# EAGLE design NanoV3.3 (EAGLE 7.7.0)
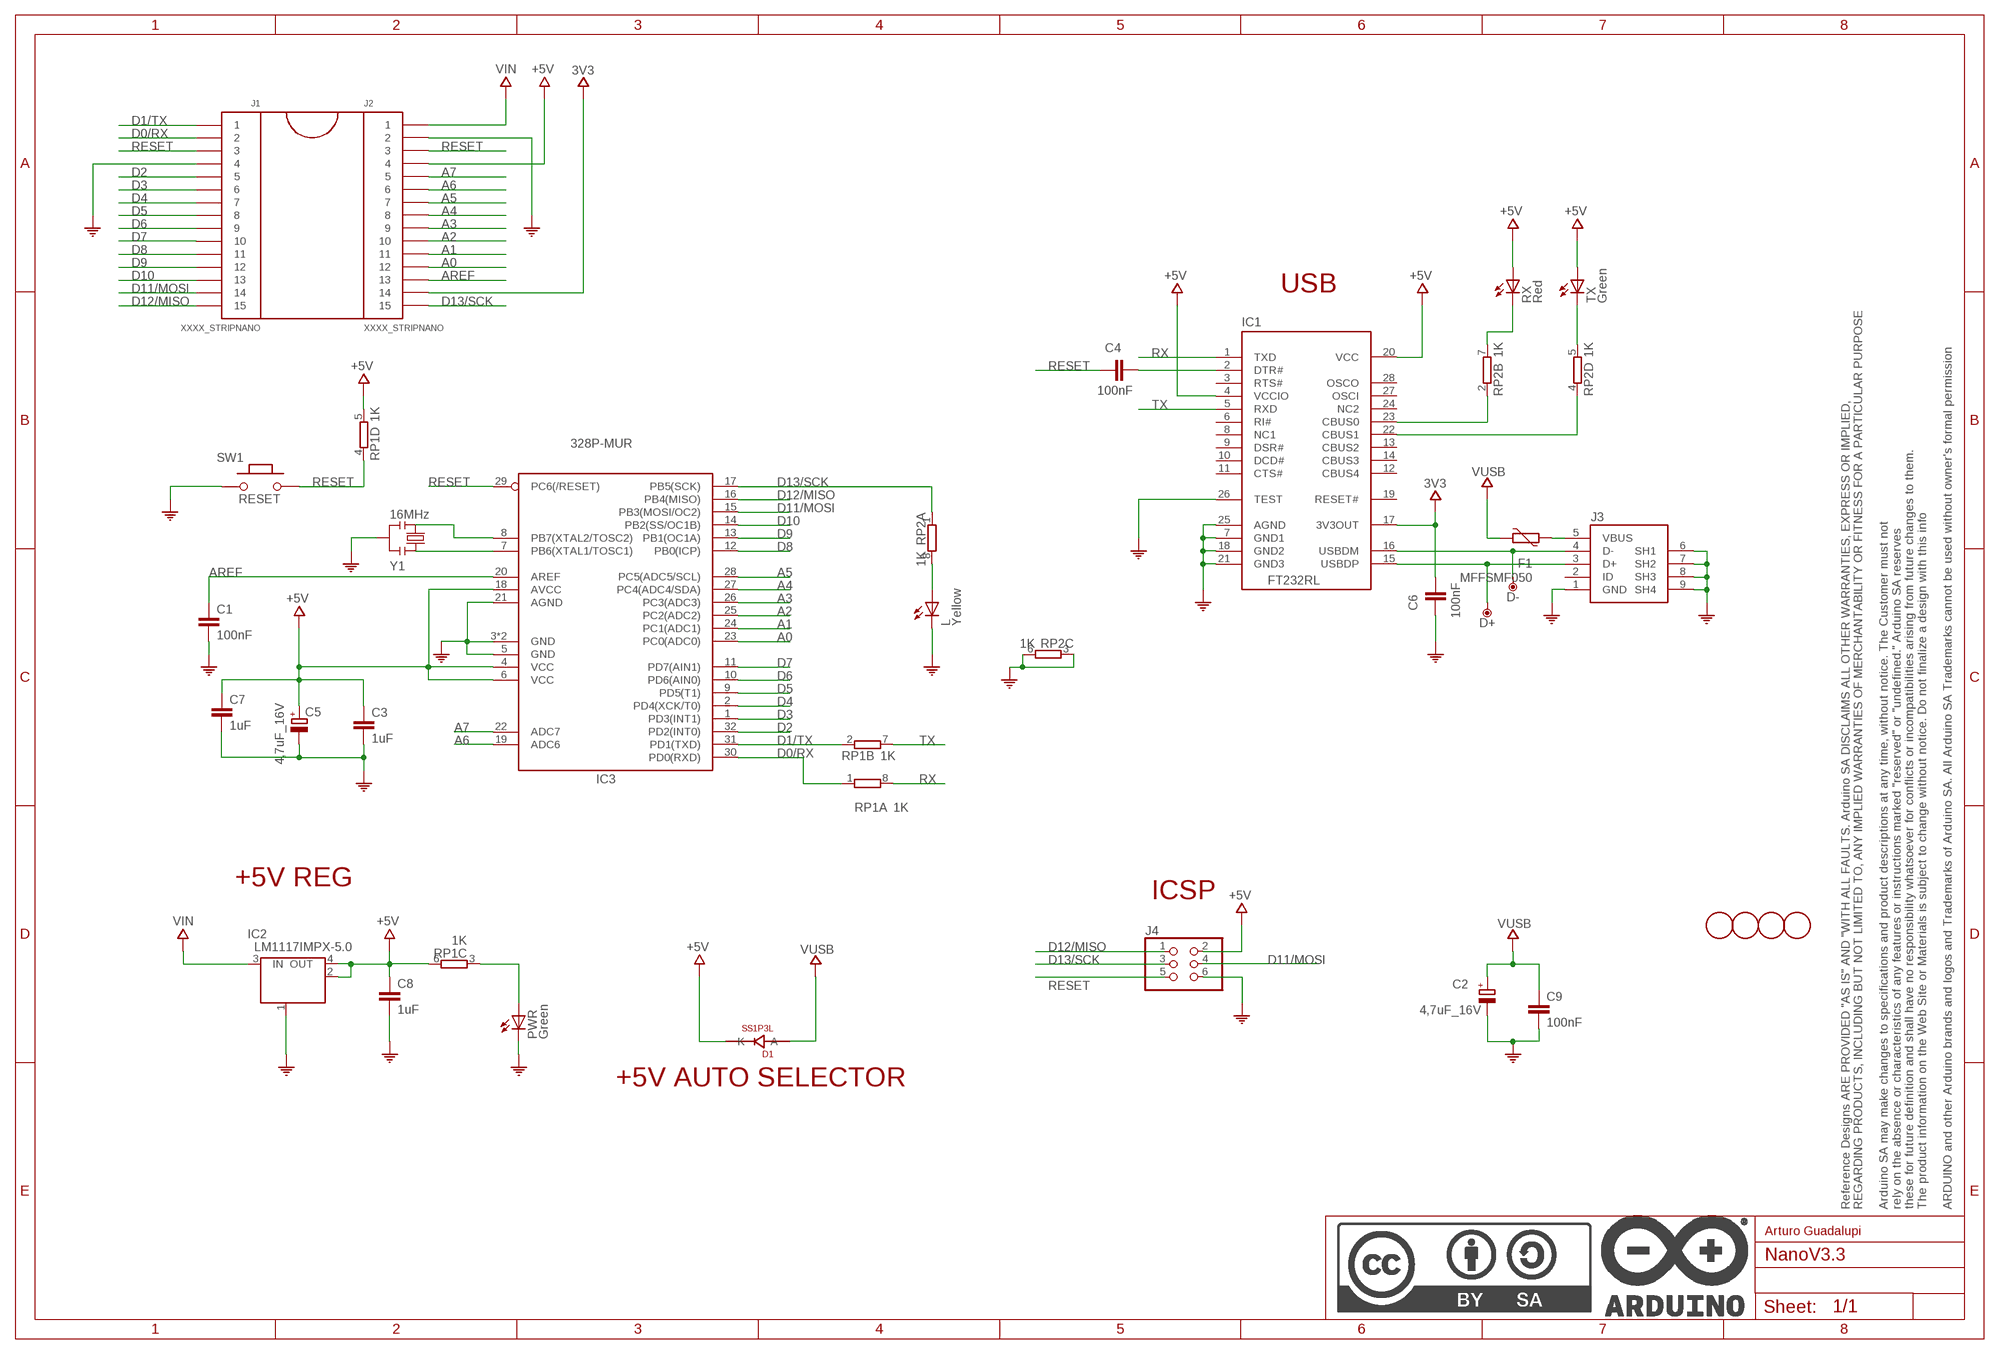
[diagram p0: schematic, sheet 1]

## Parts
C1  100nF  0015_100NF_0603  [C0603-ROUND]
C2  4,7uF_16V  0833_TAJA475MO16RNJ  [TAN-A]
C3  1uF  0006_1UF_0603/GRM188R61E105KA12D  [C0603-ROUND]
C4  100nF  0015_100NF_0603  [C0603-ROUND]
C5  4,7uF_16V  0833_TAJA475MO16RNJ  [TAN-A]
C6  100nF  0015_100NF_0603  [C0603-ROUND]
C7  1uF  0006_1UF_0603/GRM188R61E105KA12D  [C0603-ROUND]
C8  1uF  0006_1UF_0603/GRM188R61E105KA12D  [C0603-ROUND]
C9  100nF  0015_100NF_0603  [C0603-ROUND]
D1  SS1P3L  0025_SS1P3L-M3/84A  [DO220AAL]
D+  DNP  TPTP-1.00MM  [TP-1.00MM]
D-  DNP  TPTP-1.00MM  [TP-1.00MM]
F1  MFFSMF050  PTC  [0603-1608X90N]
FRAME1  DNP  A3-FRAME  [FRAME]
IC1  FT232RL  0226_FT232RL  [SSOP28]
IC2  LM1117IMPX-5.0  0022_LM1117IMPX-5.0  [LINEAR_SOT223]
IC3  328P-MUR  ATMEGA328P-32MUR  [VQFN32]
J1  XXXX_STRIPNANO  [HEAD15-NOSS]
J2  XXXX_STRIPNANO  [HEAD15-NOSS]
J3  0219_14850  [USB-MINI-B_2]
J4  0114_PH254-203DF118A00V  [2X03]
L  Yellow  0044_KPT-2012YC  [CHIPLED_0805]
PWR  Green  0043_KPT-2012SGC  [CHIPLED_0805]
RP1  1K  0005_064R_1K_/_CAY16-102J4LF  [CAY16]
RP2  1K  0005_064R_1K_/_CAY16-102J4LF  [CAY16]
RX  Red  0181_KTP-2012SURCK  [CHIPLED_0805]
SW1  RESET  0173_IT-1185AP1C-160G-G_T&R  [SMD_157SW]
TX  Green  0043_KPT-2012SGC  [CHIPLED_0805]
U$4  DNP  FIDUCIAL-1.5MM  [FD-1-1.5]
U$5  DNP  FIDUCIAL-1.5MM  [FD-1-1.5]
U$53  DNP  FIDUCIAL-1.5MM  [FD-1-1.5]
U$54  DNP  FIDUCIAL-1.5MM  [FD-1-1.5]
Y1  16MHz  0011_CSTCE16M0V53-R0  [RESONATOR]

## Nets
3V3: C6.2 IC1.17(3V3OUT) J2.14
+5V: C3.1 C5.1(+) C7.1 C8.1 D1.P$1(K) IC1.4(VCCIO) IC1.20(VCC) IC2.2(OUT) IC2.4(OUT) IC3.4(VCC) IC3.6(VCC) IC3.18(AVCC) J2.4 J4.2 RP1.5 RP1.6 RX.A TX.A
A0: IC3.23(PC0(ADC0)) J2.12
A1: IC3.24(PC1(ADC1)) J2.11
A2: IC3.25(PC2(ADC2)) J2.10
A3: IC3.26(PC3(ADC3)) J2.9
A4: IC3.27(PC4(ADC4/SDA)) J2.8
A5: IC3.28(PC5(ADC5/SCL)) J2.7
A6: IC3.19(ADC6) J2.6
A7: IC3.22(ADC7) J2.5
AREF: C1.1 IC3.20(AREF) J2.13
COM: C1.2 C2.2(-) C3.2 C5.2(-) C6.1 C7.2 C8.2 C9.2 IC1.7(GND1) IC1.18(GND2) IC1.21(GND3) IC1.25(AGND) IC1.26(TEST) IC2.1(GND/ADJ) IC3.3(GND) IC3.5(GND) IC3.21(AGND) IC3.33(GND) J1.4 J2.2 J3.1(GND) J3.6(SH1) J3.7(SH2) J3.8(SH3) J3.9(SH4) J4.6 L.C PWR.C RP2.3 RP2.6 SW1.1 Y1.2
D0/RX: IC3.30(PD0(RXD)) J1.2 RP1.1
D1/TX: IC3.31(PD1(TXD)) J1.1 RP1.2
D2: IC3.32(PD2(INT0)) J1.5
D3: IC3.1(PD3(INT1)) J1.6
D4: IC3.2(PD4(XCK/T0)) J1.7
D5: IC3.9(PD5(T1)) J1.8
D6: IC3.10(PD6(AIN0)) J1.9
D7: IC3.11(PD7(AIN1)) J1.10
D8: IC3.12(PB0(ICP)) J1.11
D9: IC3.13(PB1(OC1A)) J1.12
D10: IC3.14(PB2(SS/OC1B)) J1.13
D11/MOSI: IC3.15(PB3(MOSI/OC2)) J1.14 J4.4
D12/MISO: IC3.16(PB4(MISO)) J1.15 J4.1
D13/SCK: IC3.17(PB5(SCK)) J2.15 J4.3 RP2.1
N$1: IC3.8(PB7(XTAL2/TOSC2)) Y1.3
N$2: IC3.7(PB6(XTAL1/TOSC1)) Y1.1
N$3: PWR.A RP1.3
N$4: C4.2 IC1.2(DTR#)
N$5: D+.X IC1.15(USBDP) J3.3(D+)
N$6: D-.X IC1.16(USBDM) J3.4(D-)
N$7: L.A RP2.8
N$8: IC1.23(CBUS0) RP2.2
N$9: IC1.22(CBUS1) RP2.4
N$11: RP2.5 TX.C
N$26: F1.2 J3.5(VBUS)
N$29: RP2.7 RX.C
RESET: C4.1 IC3.29(PC6(/RESET)) J1.3 J2.3 J4.5 RP1.4 SW1.2
RX: IC1.1(TXD) RP1.8
TX: IC1.5(RXD) RP1.7
VIN: IC2.3(IN) J2.1
VUSB: C2.1(+) C9.1 D1.P$2(A) F1.1
Unconnected: IC1.3(RTS#) IC1.6(RI#) IC1.8(NC1) IC1.9(DSR#) IC1.10(DCD#) IC1.11(CTS#) IC1.12(CBUS4) IC1.13(CBUS2) IC1.14(CBUS3) IC1.19(RESET#) IC1.24(NC2) IC1.27(OSCI) IC1.28(OSCO) J3.2(ID)

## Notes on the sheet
- USB
- +5V REG
- ICSP
- +5V AUTO SELECTOR
- Arturo Guadalupi

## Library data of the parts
C1 C4 C6 C9 = Condensatori:0015_100NF_0603: 100nF 0603 50V; CASE: 0603; MONTHLY_USAGE: _____; PART_NUMBER: cl10b104kbnc; PRICE: _____; SUPPLIER: _____; TYPE: Condensatori
C2 C5 = Condensatori:0833_TAJA475MO16RNJ: 4,7uF; CASE: Case_A_(1206); MONTHLY_USAGE: _____; PART_NUMBER: TAJA475MO16RNJ; PRICE: _____; SUPPLIER: _____; TYPE: Condensatori
C3 C7 C8 = Condensatori:0006_1UF_0603/GRM188R61E105KA12D: 1uF 0603; CASE: 0603; MONTHLY_USAGE: _____; PART_NUMBER: 1uF_0603/GRM188R61E105KA12D; PRICE: _____; SUPPLIER: _____; TYPE: Condensatori
D1 = Diodi:0025_SS1P3L-M3/84A: 1A 30V Schottky Barrier Rectifiers -SS1P3L-M3/84A; CASE: SMP; MONTHLY_USAGE: _____; PART_NUMBER: SS1P3L-M3/84A; PRICE: _____; SUPPLIER: _____; TYPE: Diodi
D+ D- = Arduino-utility:TP: Testpoint; DATASHEET: DNP; DISTRIBUTOR-LINK: DNP; DISTRIBUTOR-PN: DNP; MANUFACTURER: DNP; MANUFACTURER-PN: DNP
F1 = Arduino-rcl:PTC: SMD PTC; DATASHEET: http://www.bourns.com/docs/Product-Datasheets/mffsmf.pdf; DISTRIBUTOR-LINK: http://www.digikey.com/product-detail/en/bourns-inc/MF-FSMF050X-2/MF-FSMF050X-2CT-ND/2039389; DISTRIBUTOR-PN: MF-FSMF050X-2CT-ND; MANUFACTURER: Bourns Inc; MANUFACTURER-PN: MF-FSMF050X-2
FRAME1 = Arduino-utility:A3-FRAME; CODE-ARDUINO: DNP; DATASHEET: DNP; DISTRIBUTOR-LINK: DNP; DISTRIBUTOR-PN: DNP; MANUFACTURER: DNP; MANUFACTURER-PN: DNP; NOTE: DNP
IC1 = IntegratedCircuits:0226_FT232RL: USB to serial UART interface -FT232RL; CASE: SSOP28; MONTHLY_USAGE: _____; PART_NUMBER: FT232RL; PRICE: _____; SUPPLIER: _____; TYPE: Circuito_Integrato
IC2 = IntegratedCircuits:0022_LM1117IMPX-5.0: Low-dropout linear regulator 5V -LM1117IMPX-5.0; CASE: SOT223; MONTHLY_USAGE: _____; PART_NUMBER: LM1117IMPX-5.0; PRICE: _____; SUPPLIER: _____; TYPE: Circuito_Integrato
IC3 = Arduino-ucs&SoCs:ATMEGA328P-32: 8-bit Microcontroller with 32KBytes In-System Programmable Flash ATMEGA328P-AU; DATASHEET: http://www.atmel.com/images/Atmel-8271-8-bit-AVR-Microcontroller-ATmega48A-48PA-88A-88PA-168A-168PA-328-328P_datasheet_Complete.pdf; DISTRIBUTOR-LINK: https://www.digikey.it/product-detail/it/microchip-technology/ATMEGA328P-MUR/ATMEGA328P-MURCT-ND/3440953; DISTRIBUTOR-PN: ATMEGA328P-MURCT-ND; MANUFACTURER: ATMEL; MANUFACTURER-PN: ATMEGA328P-MUR
J1 J2 = Connettori:XXXX_STRIPNANO: Strip passo 2,54 a 15 pin per Arduino Nano; VALUE: Strip15pin
J3 = Connettori:0219_14850: Usb-Mini F 90 Smd; MONTHLY_USAGE: _____; PART_NUMBER: 14850; PRICE: _____; SUPPLIER: _____; TYPE: Connettori; VALUE: USB-mini-90 -SMD
J4 = Connettori:0114_PH254-203DF118A00V: 3x2 M V h 8,5 mm p2,54; MONTHLY_USAGE: _____; PART_NUMBER: PH254-203DF118A00V; PRICE: _____; SUPPLIER: _____; TYPE: Connettori; VALUE: ICSP
L = Opto:0044_KPT-2012YC: LED YELLOW - SMD - 0805; MONTHLY_USAGE: _____; PART_NUMBER: KPT-2012YC; PRICE: _____; SUPPLIER: _____; TYPE: Opto
PWR TX = Opto:0043_KPT-2012SGC: LED GREEN - SMD-0805; MONTHLY_USAGE: _____; PART_NUMBER: KPT-2012SGC; PRICE: _____; SUPPLIER: _____; TYPE: Opto
RP1 RP2 = Resistenze:0005_064R_1K_/_CAY16-102J4LF: 1K 064R; CASE: SMD_3,2x1,6; MONTHLY_USAGE: _____; PART_NUMBER: 064R_1K_/_CAY16-102J4LF; PRICE: _____; SUPPLIER: _____; TYPE: Resistenze
RX = Opto:0181_KTP-2012SURCK: LED RED - SMD - 0805; MONTHLY_USAGE: _____; PART_NUMBER: KTP-2012SURCK; PRICE: _____; SUPPLIER: _____; TYPE: Opto
SW1 = Switches:0173_IT-1185AP1C-160G-G_T&R: Pushbutton 4x3 SMD H2,5mm; MONTHLY_USAGE: _____; PART_NUMBER: IT-1185AP1C-160G-G_T&R; PRICE: _____; SUPPLIER: _____; TYPE: Switches; VALUE: 157SW
U$4 U$5 U$53 U$54 = Arduino-utility:FIDUCIAL: Fiducial mount; DATASHEET: DNP; DISTRIBUTOR-LINK: DNP; DISTRIBUTOR-PN: DNP; MANUFACTURER: DNP; MANUFACTURER-PN: DNP
Y1 = Cristalli:0011_CSTCE16M0V53-R0: 16Mhz - SMD; MONTHLY_USAGE: _____; PART_NUMBER: CSTCE16M0V53-R0; PRICE: _____; SUPPLIER: _____; TYPE: Cristalli; VALUE: CSTCE16M0V53-R0

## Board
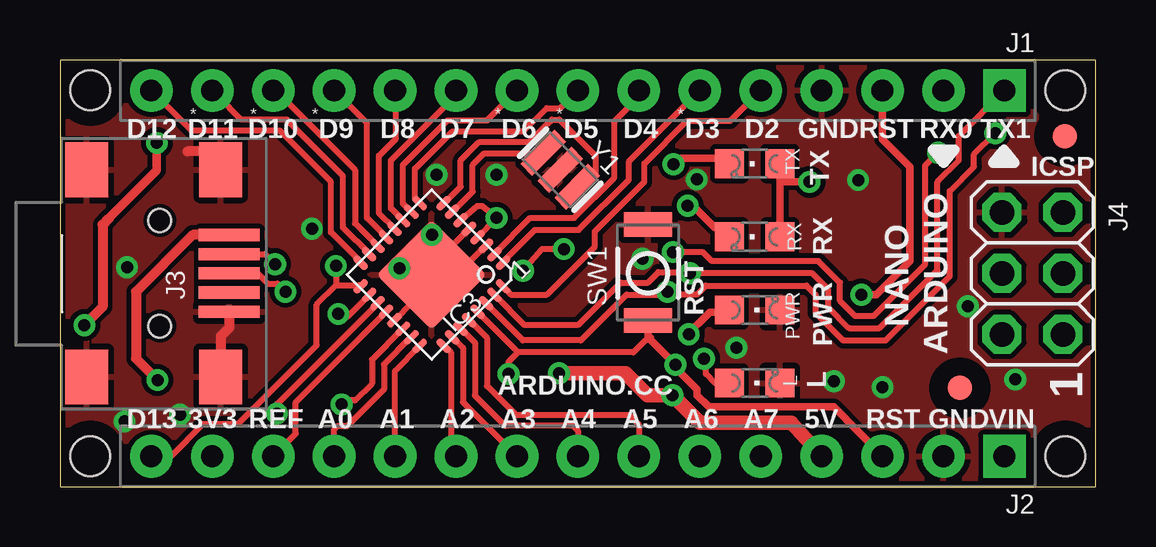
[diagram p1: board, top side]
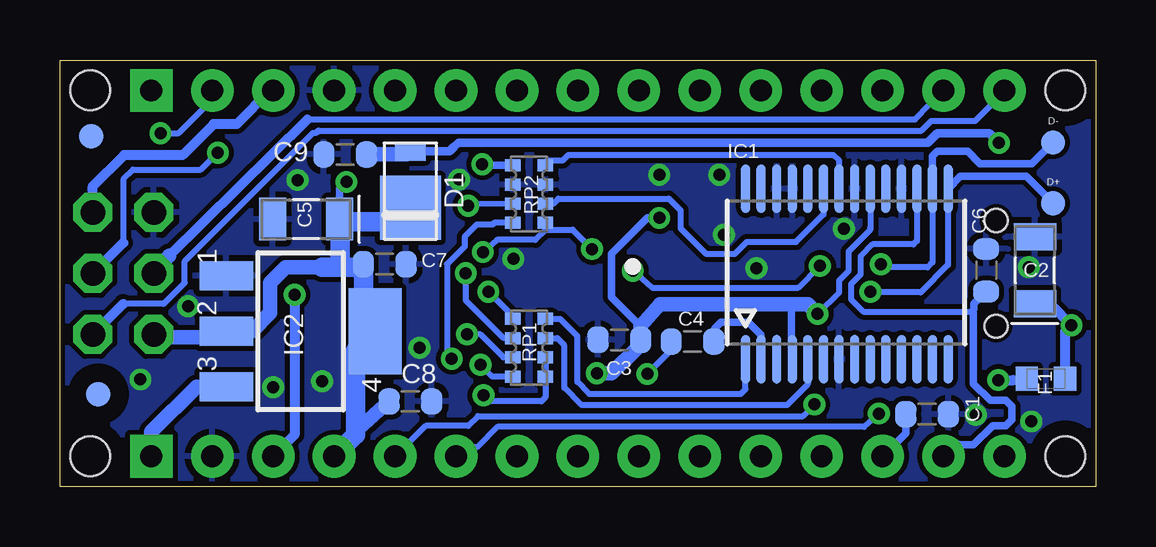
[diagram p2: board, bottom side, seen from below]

Size 43.18 x 17.78 mm. Coordinates in mm from the lower left corner, seen from the top.
Outline: 0,17.78 0,0 43.18,0 43.18,17.78 0,17.78
Copper layers (1*16): Top 0.035mm / dielectric 1.5mm / Bottom 0.035mm
Design rules "default *": minimum track width 10mil, minimum drill 16mil, track to track 8mil, track to pad 8mil, pad to pad 8mil, via to via 8mil, smd to smd 8mil, copper to edge 8mil, drill to drill 8mil, minimum pad ring 12mil, minimum via ring 8mil, stop-mask expansion 0mil, vias tented up to drill 24mil, thermal gap 10mil
Holes 1.65 mm at 1.27,16.51 1.27,1.27 41.91,1.27 41.91,16.51
tRestrict: area 0.1,15.4 to 2.4,17.7; area 40.8,0.1 to 43.1,2.4; area 0.1,0.1 to 2.4,2.4; area 40.8,15.4 to 43.1,17.7
bRestrict: area 0.1,0.1 to 2.4,2.4; area 0.1,15.4 to 2.4,17.7; area 40.8,15.4 to 43.1,17.7; area 40.8,0.1 to 43.1,2.4

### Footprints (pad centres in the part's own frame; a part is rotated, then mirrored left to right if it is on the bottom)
C0603-ROUND = smd 0.898 x 1.1: 1 -0.889,0; 2 0.889,0
TAN-A = smd 1.118 x 1.778: 1 0,0; 2 2.794,0
DO220AAL = smd 2.667 x 2.54: P$1 -0.7,0 | smd 0.762 x 1.27: P$2 1.65,0
TP-1.00MM = smd 1 x 1 bottom: X 0,0
0603-1608X90N = smd 0.95 x 1: 1 -0.8,0; 2 0.8,0
SSOP28 = smd 0.381 x 2.032: 1 0,0; 2 0.65,0; 3 1.3,0; 4 1.95,0; 5 2.6,0; 6 3.25,0; 7 3.9,0; 8 4.55,0; 9 5.2,0; 10 5.85,0; 11 6.5,0; 12 7.15,0; 13 7.8,0; 14 8.45,0; 15 8.45,7.112; 16 7.8,7.112; 17 7.15,7.112; 18 6.5,7.112; 19 5.85,7.112; 20 5.2,7.112; 21 4.55,7.112; 22 3.9,7.112; 23 3.25,7.112; 24 2.6,7.112; 25 1.95,7.112; 26 1.3,7.112; 27 0.65,7.112; 28 0,7.112
LINEAR_SOT223 = smd 1.219 x 2.235: 1 -2.311,-3.099; 2 0,-3.099; 3 2.311,-3.099 | smd 3.6 x 2.2: 4 0,3.099
VQFN32 = smd 0.7 x 0.28: 1 -2.45,1.75; 2 -2.45,1.25; 3 -2.45,0.75; 4 -2.45,0.25; 5 -2.45,-0.25; 6 -2.45,-0.75; 7 -2.45,-1.25; 8 -2.45,-1.75; 17 2.45,-1.75; 18 2.45,-1.25; 19 2.45,-0.75; 20 2.45,-0.25; 21 2.45,0.25; 22 2.45,0.75; 23 2.45,1.25; 24 2.45,1.75 | smd 0.28 x 0.7: 9 -1.75,-2.45; 10 -1.25,-2.45; 11 -0.75,-2.45; 12 -0.25,-2.45; 13 0.25,-2.45; 14 0.75,-2.45; 15 1.25,-2.45; 16 1.75,-2.45; 25 1.75,2.45; 26 1.25,2.45; 27 0.75,2.45; 28 0.25,2.45; 29 -0.25,2.45; 30 -0.75,2.45; 31 -1.25,2.45; 32 -1.75,2.45 | smd 3.254 x 3.254: 33 0,0
HEAD15-NOSS = drill 0.914 pad 1.778 square: 1 0,0 | drill 0.914 pad 1.778: 2 2.54,0; 3 5.08,0; 4 7.62,0; 5 10.16,0; 6 12.7,0; 7 15.24,0; 8 17.78,0; 9 20.32,0; 10 22.86,0; 11 25.4,0; 12 27.94,0; 13 30.48,0; 14 33.02,0; 15 35.56,0
USB-MINI-B_2 = smd 0.508 x 2.54: 1 0,0; 2 0.8,0; 3 1.6,0; 4 2.4,0; 5 3.2,0 | smd 2.286 x 1.778: 6 -2.717,5.948; 7 -2.717,0.36; 8 5.918,0.36; 9 5.918,5.948 | hole 0.95: -0.6,2.9; 3.8,2.9
2X03 = drill 1.016 pad 1.55 octagon: 1 -2.54,-1.27; 2 -2.54,1.27; 3 0,-1.27; 4 0,1.27; 5 2.54,-1.27; 6 2.54,1.27
CHIPLED_0805 = smd 1.2 x 1.2: A 0,-1.05; C 0,1.05
CAY16 = smd 0.5 x 0.65: 1 -1.2,-0.675; 2 -0.4,-0.675; 3 0.4,-0.675; 4 1.2,-0.675; 5 1.2,0.675; 6 0.4,0.675; 7 -0.4,0.675; 8 -1.2,0.675
SMD_157SW = smd 1.016 x 1.981: 1 0,0; 2 4,0
FD-1-1.5 = smd 1.016 x 1.016: P$1 0,0
RESONATOR = smd 0.7 x 2: 1 -1,0; 2 0,0; 3 1,0

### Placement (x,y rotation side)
C1  7.04,3.02 0 bottom
C2  2.54,7.62 90 bottom
C3  19.86,6.12 180 bottom
C4  16.81,6.05 0 bottom
C5  31.52,11.15 180 bottom
C6  4.57,9.02 270 bottom
C7  29.64,9.27 0 bottom
C8  28.57,3.56 0 bottom
C9  31.29,13.84 180 bottom
D1  28.57,12.32 90 bottom
D+  1.78,11.81 0 top
D-  1.78,14.35 0 top
F1  2.08,4.5 180 bottom
FRAME1  0,0 0 top
IC1  14.61,5.31 0 bottom
IC2  33.15,6.48 270 bottom
IC3  15.49,8.84 225 top
J1  39.37,16.51 180 top
J2  39.37,1.27 180 top
J3  7.06,7.29 90 top
J4  40.54,8.89 90 top
L  28.96,4.32 270 top
PWR  28.96,7.37 270 top
RP1  23.62,5.79 270 bottom
RP2  23.62,12.19 90 bottom
RX  28.96,10.41 90 top
SW1  24.51,10.92 270 top
TX  28.96,13.46 90 top
U$4  37.52,4.11 270 top
U$5  41.88,14.61 0 top
U$53  41.58,3.86 90 bottom
U$54  41.88,14.61 90 bottom
Y1  20.85,13.21 315 top

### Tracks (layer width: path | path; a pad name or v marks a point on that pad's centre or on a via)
3V3
  Bottom 0.254: IC1.17 7.46,10.24 7.6,10.1 9.31,10.1 9.31,10.09 9.8,9.6 9.8,8.85 10.2,8.45 10.2,7.8 9.7,7.3 5.18,7.3 5.08,7.4
  Bottom 0.305: 4.6,8.15 C6.2 5.08,7.62 5.08,7.4 | 5.71,1.78 5.84,1.78 J2.14 5.87,1.75 5.1,1.75 4.3,2.55 3.75,2.55 3.5,2.8 3.5,3.35 3.75,3.6 4.4,3.6 5.1,4.3 5.1,7.22 5.18,7.3
+5V  (via drill 0.5, 0.5 pad 0.91)
  Top 0.254: IC3.18 12.88,7.98 12,7.1 11.7,7.1 v11.6,7.2 | IC3.4 17.4,10.4 v18.2,11.2 17.6,11.7 17.4,11.7 IC3.6
  Top 0.305: TX.A 30.01,12.7 | 30.01,12.7 RX.A | v31.24,12.7 30.01,12.7
  Top 0.61: v20.8,4.72 23.57,4.72 24.49,3.81 v25.53,3.81 26.67,2.67 30.48,2.67 J2.4
  Bottom 0.254: 12.7,5.38 IC1.4 | v25.53,3.81 25.27,3.56 23.11,3.56 22.95,3.72 RP1.5 RP1.6 | 18.1,7.55 18.16,7.59 | IC1.20 9.4,10.71 | v11.6,7.2 10.7,8.1 10.7,8.6 10.3,9 10.3,9.81 9.4,10.71 | 9.4,10.71 9.4,10.8
  Bottom 0.305: 29.34,4.95 29.34,5.77 IC2.4 | C5.1 31.52,12.42 v31.24,12.7 | 12.7,5.38 12.7,7.39 12.6,7.59 | 18.97,6.68 20,7.71 20.01,7.71 20.2,7.9 20.2,9.7 18.7,11.2 v18.2,11.2
  Bottom 0.406: IC2.2 36.37,6.35 | 30.61,7.37 30.61,7.04 30.45,6.88 | 30.45,6.88 IC2.4 | 30.12,7.21 30.45,6.88 | 31.42,11.05 C5.1
  Bottom 0.61: 36.37,6.35 36.96,6.35 37.08,6.22 38.73,6.22 38.86,6.35 J4.2 | IC2.2 35.18,6.48 34.42,7.24 34.42,8.51 33.78,9.14 32.26,9.14 | D1.P$1 28.77,11.62 29.34,11.05 | C8.1 30.73,2.41 30.86,2.41 | 20.8,4.75 v20.8,4.72 20.19,4.72 19.07,5.84 C3.1 18.97,6.68 18.16,7.59 12.6,7.59 11.99,7.59 v11.6,7.2
  Bottom 0.813: IC2.4 30.86,5.66 30.86,2.41 30.86,2.16 J2.4 | 29.34,11.05 31.42,11.05 | 30.12,7.21 30.53,7.37 C7.1 30.66,9.14 31.5,9.14 | 32.26,9.14 31.5,9.14 | 31.5,9.14 31.5,11.12 C5.1
A0
  Top 0.254: J2.12 11.43,2.39 11.58,2.54 11.99,2.54 13.5,4.05 13.5,5.1 14.62,6.22 IC3.23
A1
  Top 0.254: J2.11 13.97,4.84 IC3.24
A2
  Top 0.254: IC3.25 16.03,5.87 16.3,5.6 16.3,1.48 J2.10
A3
  Top 0.254: IC3.26 16.38,6.22 16.8,5.8 16.8,3.52 J2.9
A4
  Top 0.254: J2.8 21.59,2.34 21.39,2.54 18.56,2.54 17.3,3.8 17.3,6 16.72,6.58 IC3.27
A5
  Top 0.254: J2.7 24.13,2.59 23.72,3 19,3 17.8,4.2 17.8,6.2 17.07,6.93 IC3.28
A6  (via drill 0.5 pad 0.81)
  Top 0.254: IC3.19 9.04,3.44 v9.04,3.05
  Bottom 0.254: J2.6 26.29,1.65 25.78,1.65 24.94,2.49 9.65,2.49 v9.04,3.05
A7  (via drill 0.5 pad 0.81)
  Top 0.254: 11.73,3.4 v11.73,3.43 11.91,3.6 12.3,3.6 13,4.3 13,5.3 14.28,6.58 IC3.22
  Bottom 0.254: J2.5 27.94,2.54 26.16,2.54 25.76,2.95 12.22,2.95 v11.73,3.43
AREF
  Top 0.254: J2.13 9.83,2.21 9.83,3.53 IC3.20
  Bottom 0.305: C1.1 7.92,2.24 J2.13
COM  (via drill 0.5, 0.5 pad 0.81, 0.5 pad 0.91)
  Top 0.254: IC3.5 16.1,9.8 | IC3.3 17.74,10.04 16.8,9.1 | IC3.21 14.7,7.7 14.7,8.04 | 14.7,8.04 IC3.33 16.1,9.45 16.1,9.8 | 16.1,9.8 15.7,9.8 v15.5,10.5 | 14.7,8.04 14.7,8.55 v14.15,9.1
  Top 0.305: 16.8,9.1 16.4,9.1 v15.5,10.5
  Top 0.406: J3.1 7.06,6.63 6.71,6.27 J3.7 | J3.8 6.7,13.97 5.31,13.97
  other vias: 39.83,4.47 33.27,12.78 26.54,12.8 28.19,5.79 32.26,4.39 34.29,4.14 37.85,7.52 24.28,9.5 2.69,2.72 2.79,9.14 15.7,13 18.2,13 10.5,10.75 5,3
  pour Top (isolate 0.203): 0.25,17.53 46.23,17.65 46.23,0.38 0.25,0.25
  pour Bottom (isolate 0.203): 0.25,17.53 44.83,17.65 44.83,0.38 0.25,0.25
D0/RX  (via drill 0.5, 0.5 pad 0.81)
  Top 0.254: v25.32,8.13 25.07,8 23.62,8 21.72,6.1 21.71,6.1 19.3,6.1 IC3.30 | v38.99,14.73 38.1,13.84 38.1,13.34 37.08,12.32 37.08,8.76 34.42,6.1 32.64,6.1 31.5,7.24 31.5,8 31.11,8.38 26.92,8.38 26.54,8 25.45,8 v25.32,8.13 | 25.4,8.13 v25.32,8.13
  Bottom 0.254: J1.2 36.83,16.13 38.23,14.73 v38.99,14.73 | RP1.1 24.3,7.1 v25.32,8.13
D1/TX  (via drill 0.5)
  Top 0.254: J1.1 37.47,14.61 37.47,13.59 36.58,12.7 36.58,9.02 34.16,6.6 32.89,6.6 32,7.49 32,8.26 31.37,8.89 v26.26,8.89 26.21,8.94 24.94,8.94 24.51,8.51 23.37,8.51 21.59,6.73 19.37,6.73 IC3.31
  Bottom 0.254: RP1.2 24.68,6.19 26.26,7.77 v26.26,8.89
D2
  Top 0.254: J1.5 27.94,15.24 26.14,15.24 24.36,13.46 24.36,12.7 22.3,10.64 22.3,10 20.3,8 18.8,8 IC3.32
D3
  Top 0.254: J1.6 23.7,13.54 23.7,12.8 23.71,12.79 21.62,10.7 19.8,10.7 18.46,9.36 IC3.1
D4
  Top 0.254: J1.7 24.13,16.26 23.09,15.21 23.09,12.85 21.44,11.2 19.6,11.2 18.11,9.71 IC3.2
D5
  Top 0.254: J1.8 20.85,15.77 20.3,15.77 19.33,14.81 16.36,14.81 14.8,13.25 14.8,12 IC3.9
D6
  Top 0.254: J1.9 17.8,15.27 16.15,15.27 14.3,13.41 14.3,11.8 IC3.10 | IC3.10
D7
  Top 0.254: IC3.11 13.8,11.6 13.8,13.6 16.51,16.31 J1.10
D8
  Top 0.254: IC3.12 13.94,10.76 13.3,11.4 13.3,13.8 14,14.5 14,16.48 J1.11
D9
  Top 0.254: IC3.13 13.59,10.41 12.8,11.2 12.8,15.14 J1.12
D10
  Top 0.254: 13.23,10.07 IC3.14 12.3,10.97 12.3,13.2 8.99,16.51 J1.13
D11/MOSI
  Top 0.254: J1.14 7.07,15.79 7.07,15.78 7.55,15.29 9.45,15.29 11.8,12.94 11.8,10.8 12.88,9.72 IC3.15
  Bottom 0.254: 32.87,15.29 7.54,15.29 J1.14
  Bottom 0.406: 38.63,9.63 32.87,15.29
  Bottom 0.61: J4.4 38.63,9.63
D12/MISO
  Top 0.254: J1.15 5.49,14.83 9.17,14.83 11.3,12.7 11.3,10.6 12.52,9.38 IC3.16
  Bottom 0.254: 40.54,7.62 38.86,7.62 37.97,8.51 37.97,9.4 32.64,14.73 32.51,14.73 32.41,14.83 7.26,14.83 6.86,15.24 5.03,15.24 3.81,16.46 J1.15
  Bottom 0.406: 40.54,7.62 J4.1
D13/SCK  (via drill 0.5, 0.5 pad 0.81, 0.5 pad 0.91)
  Top 0.254: v25.55,9.78 26.8,9.78 27.18,9.4 31.62,9.4 32.51,8.51 32.51,7.75 33.15,7.11 33.91,7.11 36.07,9.27 36.07,13.39 v36.6,13.92 | 11.5,8.4 10.7,7.6 10.7,5.9 7.4,2.6 5.95,2.6 4.65,1.3 3.84,1.3 J2.15 | 11.5,8.4 12.47,8.4 IC3.17 | v21,9.9 20.1,9.9 v19.3,9 | v11.5,9.2 11.5,8.4
  Bottom 0.254: 40.54,10.16 40.54,12.8 40.13,13.21 37.31,13.21 v36.6,13.92 | RP2.1 22.95,10.71 | 22.95,10.71 23.37,10.29 24.97,10.29 v25.55,9.78 | 22.95,10.71 21.81,10.71 v21,9.9 | v19.3,9 18.5,8.3 12.4,8.3 v11.5,9.2
  Bottom 0.406: 40.54,10.16 J4.3
N$1
  Top 0.254: Y1.3 21.54,12.24 22.33,13.03 22.33,13.79 20.82,15.3 20.5,15.3 20.34,15.14 19.56,14.35 17.45,14.35 16.7,13.6 16.7,12.5 16.01,11.81 IC3.8
N$2
  Top 0.254: Y1.1 19.89,13.89 17.68,13.89 17.2,13.41 17.2,12.3 16.36,11.46 IC3.7
N$3  (via drill 0.5)
  Top 0.305: PWR.A 27.65,7.27 27.09,7.27 26.04,6.22 26.16,6.3 v26.21,6.35
  Bottom 0.254: v26.21,6.35 25.65,6.35 24.7,5.39 RP1.3
N$4
  Bottom 0.305: C4.2 15.88,6.1 15.88,6.6 15.62,6.86 14.48,6.86 13.96,6.33 IC1.2
N$5  (via drill 0.5 pad 0.81)
  Top 0.254: J3.3 8.23,8.89 8.66,8.46 9.07,8.46 v9.4,8.13 | J3.3
  Bottom 0.254: 6.15,12.45 6.16,12.43 6.16,12.32 6.16,9.24 7.3,8.1 9.37,8.1 v9.4,8.13
  Bottom 0.305: D+.X 2.9,12.93 5.65,12.93 IC1.15
  Bottom 0.356: IC1.15 6.16,12.32
N$6  (via drill 0.5 pad 0.81)
  Top 0.254: J3.4 8.55,9.69 v8.97,9.27
  Bottom 0.254: 6.79,12.45 6.81,12.43 6.81,9.35 7.01,9.14 8.84,9.14 v8.97,9.27
  Bottom 0.305: IC1.16 6.8,13.77 6.6,13.97 5.33,13.97 4.83,13.46 2.67,13.46 D-.X
  Bottom 0.356: IC1.16 6.81,12.43
N$7  (via drill 0.5 pad 0.81)
  Top 0.254: 27.92,4.32 27.3,4.32 26.92,4.7 26.95,5.08 v26.85,5.33
  Top 0.305: L.A 28.04,4.2 27.92,4.32
  Bottom 0.254: v26.85,5.33 27.05,5.61 27.05,9.27 26.31,10.01 26.31,10.41 25.81,10.92 25.15,10.92 25.08,10.99 RP2.8
N$8
  Bottom 0.254: RP2.2 22.93,11.81 22.59,11.81 22.4,12 17.8,12 17.3,11.5 17.3,10.75 16.25,9.7 15.05,9.7 14.55,10.2 12.5,10.2 11.35,11.35 IC1.23
  Bottom 0.305: IC1.23
N$9
  Bottom 0.254: IC1.22 10.71,13.6 10.95,13.82 22,13.82 22,13.81 22.23,13.59 22.88,13.59 RP2.4
N$11  (via drill 0.5 pad 0.81)
  Top 0.305: TX.C 27.88,13.69 25.88,13.69 25.78,13.59 v25.58,13.44
  Bottom 0.305: RP2.5 25.53,13.39 v25.58,13.44
N$26  (via drill 0.5)
  Top 0.406: J3.5 5.54,10.49 3.17,8.13 3.17,5.33 v4.06,4.45
  Bottom 0.406: v4.06,4.45 3.44,4.45 F1.2
N$29  (via drill 0.5)
  Top 0.305: RX.C 27.69,10.79 27.3,10.79 26.42,11.68 v26.16,11.71
  Bottom 0.254: RP2.7 26.04,11.78 v26.16,11.71
RESET  (via drill 0.5, 0.5 pad 0.91)
  Top 0.254: 19.09,5.6 23.9,5.6 24.4,6.1 24.64,6.1 24.64,6.22 24.51,6.22 | 17.42,7.28 IC3.29 19.09,5.6 | v18.7,4.7 18.7,5.21 19.09,5.6
  Top 0.305: J2.3 32.26,3.33 27.05,3.33 26.54,3.81 26.54,4.06 25.65,4.95 v25.65,5.08 24.64,6.1 | J1.3 34.29,14.48 35.43,13.34 35.43,9.4 34.04,8 v33.4,8 | 24.77,6.67 SW1.2 | 25.27,6.99 25.21,6.92 SW1.2 | 24.51,6.22 SW1.2
  Bottom 0.254: J1.3 34.42,16.51 | RP1.4 25.16,4.59 v25.65,5.08 | C4.1 | 17.7,5.7 v18.7,4.7
  Bottom 0.305: C4.1 17.7,5.77 | C4.1 17.7,5.7
  Bottom 0.406: v33.4,8 33.4,2.16 J2.3 | 34.42,16.51 35.81,15.11 36.78,15.11 38.08,13.82 40.51,13.82 41.81,12.52 J4.5
RX
  Bottom 0.254: IC1.1 14.61,4.06 14.81,3.86 21.11,3.86 21.61,4.37 21.61,6.27 22.33,6.99 RP1.8
TX
  Bottom 0.254: IC1.5 12.01,4.28 12.88,3.4 21.44,3.4 22.15,4.12 22.15,5.89 22.45,6.19 RP1.7
VIN
  Bottom 0.61: IC2.3 37.49,4.17 39.37,2.29 J2.1
VUSB  (via drill 0.5)
  Top 0.356: v4.04,14.33 4.04,13.18 2.03,11.18
  Top 0.406: 2.03,11.18 1.78,10.92 1.78,7.49 v1.02,6.73
  Bottom 0.356: v4.04,14.33 4.45,14.73 6.6,14.73 7.01,14.33 26.57,14.33 26.75,14.17 26.95,13.97 D1.P$2
  Bottom 0.406: 28.83,13.84 D1.P$2 | C2.1 1.91,7.62 v1.02,6.73 1.28,6.46 F1.1
  Bottom 0.61: D1.P$2 28.7,13.84 C9.1

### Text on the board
tPlace: D12 | D11 | * | D10 | * | * | D9 | D8 | D7 | * | D6 | * | D5 | D4 | * | D3 | D2 | GND | RST | RX0 | TX1 | TX | ICSP | ARDUINO | RX | NANO | RST | PWR | L | 1 | ARDUINO.CC | D13 | 3V3 | REF | A0 | A1 | A2 | A3 | A4 | A5 | A6 | A7 | 5V | RST | GND | VIN
test-probe: NANO / TEST POINTS | 10 | 9 | 8 | 7 | 6 | 5 | 4 | 3 | 2 | GND1 | RESET | 0 | 1 | USB_D- | USB_D+ | USB_GND | ISP1_5 | ISP1_4 | ISP1_3 | USB_5V | ISP1_1 | 3V3 | AREF | A0 | A1 | A2 | A3 | A4 | A5 | A6 | A7 | 5V_REF | DC_VIN- | DC_VIN+

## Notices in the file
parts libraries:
Arduino-utility: Copyright (c) 2016-2017 Arduino LLC. All right reserved.
